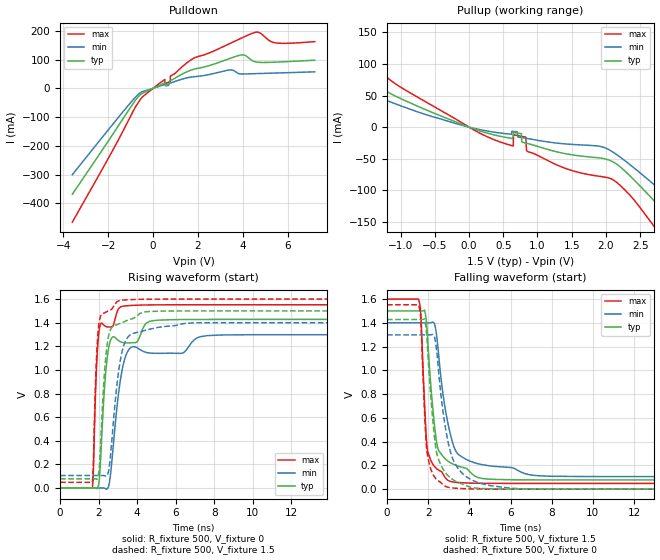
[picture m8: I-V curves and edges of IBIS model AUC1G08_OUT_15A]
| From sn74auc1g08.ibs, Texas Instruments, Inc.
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[Model]   AUC1G08_OUT_15A
Model_type  Output
Vref =   0
Rref =   2000
Cref =   15p
Vmeas =   0.75
| variable   typ   min   max
C_comp   7.20pF   2.74pF   16.84pF
| C_pullup   7.06pF   2.77pF   16.84pF
| C_pulldown   7.34pF   2.74pF   15.89pF
[Temperature Range]   40   100   -40
| Ambient temperature   25   85   -40
[Voltage range]   1.5   1.4   1.6
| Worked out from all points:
|   slope of the pulldown table from 0 to 0.225 V, typ, clamps not added: 27.2 ohm
|   slope of the pullup table from 0 to 0.225 V, typ, clamps not added: 27.6 ohm
|   rising waveform, R_fixture 500, V_fixture 0: 20-80 % time 361ps typ, 564ps min, 214ps max; typ from 0 V to 1.43 V
|   falling waveform, R_fixture 500, V_fixture 1.5: 20-80 % time 454ps typ, 736ps min, 255ps max; typ from 1.5 V to 0.078 V
|   rising waveform, R_fixture 500, V_fixture 1.5: 20-80 % time 344ps typ, 533ps min, 205ps max; typ from 0.078 V to 1.5 V
|   falling waveform, R_fixture 500, V_fixture 0: 20-80 % time 453ps typ, 701ps min, 256ps max; typ from 1.43 V to 0 V
[Pulldown]
| AUC1G08_OUT_15A
|   Voltage   I(typ)   I(min)   I(max)
-3.6V     -368.8mA   -300.6mA   -465.9mA
-570mV    -22.57mA   -15.16mA   -39.04mA
520mV     19.17mA    13.19mA    30.72mA
525mV     19.35mA    13.3mA     16.47mA
760mV     26.99mA    18.45mA    23.24mA
780mV     27.61mA    18.9mA     43.29mA
1.55V     59.04mA    37.1mA     91.54mA
3.425V    104mA      63.97mA    156.1mA
3.925V    116.2mA    49.97mA    174.5mA
4.58V     91.74mA    51.18mA    195.4mA
5.455V    91.13mA    53.24mA    158.3mA
7.2V      97.82mA    57.36mA    162.5mA
[Pullup]
| AUC1G08_OUT_15A
|   Voltage   I(typ)   I(min)   I(max)
-3.6V     253.4mA    202.6mA    313.9mA
-3.11V    208.7mA    165mA      264.9mA
-2.525V   156.9mA    121.3mA    206.3mA
-2.08V    119.5mA    90.68mA    162.1mA
80mV      -3.149mA   -2.07mA    -5.073mA
645mV     -8.448mA   -6.832mA   -29.87mA
830mV     -25.21mA   -17.58mA   -15.88mA
860mV     -25.98mA   -18.12mA   -38.83mA
2.065V    -52.94mA   -36.97mA   -81.25mA
2.79V     -126.2mA   -98.83mA   -169.6mA
3.55V     -215.2mA   -171.3mA   -279.9mA
7.2V      -643.1mA   -531.6mA   -796.6mA
[Ramp]
| AUC1G08_OUT_15A
| variable   typ   min   max
dV/dt_r   0.86/3.66E-10   0.79/5.70E-10   0.93/2.16E-10
dV/dt_f   0.86/4.64E-10   0.78/7.36E-10   0.93/2.56E-10
R_load = 500
[Rising Waveform]
| AUC1G08_OUT_15A
R_fixture =   500
C_fixture =   0
L_fixture =   0
V_fixture =   0
V_fixture_min = 0
V_fixture_max = 0
|   Time   V(typ)   V(min)   V(max)
0s        5.666nV    22.19nV    433.4pV
1.67ns    28.86uV    -4.974uV   968.1uV
1.88ns    -2.649mV   -6.943uV   995.4mV
2.035ns   79.02mV    138.4uV    1.346V
2.295ns   833.3mV    -1.097mV   1.375V
2.5ns     1.17V      7.839mV    1.363V
3.185ns   1.234V     972.6mV    1.537V
3.7ns     1.23V      1.193V     1.546V
7.63ns    1.427V     1.29V      1.552V
24.99ns   1.428V     1.298V     1.552V
[Falling Waveform]
| AUC1G08_OUT_15A
R_fixture =   500
C_fixture =   0
L_fixture =   0
V_fixture =   1.5
V_fixture_min = 1.4
V_fixture_max = 1.6
|   Time   V(typ)   V(min)   V(max)
0s        1.5V       1.4V       1.6V
1.54ns    1.5V       1.4V       1.594V
1.635ns   1.5V       1.4V       1.493V
1.83ns    1.502V     1.4V       691.6mV
1.965ns   1.293V     1.399V     325.6mV
2.42ns    384.1mV    1.279V     171.4mV
3.065ns   224.1mV    470.9mV    66.14mV
3.885ns   171.7mV    247.6mV    52.3mV
7.185ns   78.16mV    115.4mV    48.34mV
24.99ns   77.67mV    105.5mV    48.23mV
[Rising Waveform]
| AUC1G08_OUT_15A
R_fixture =   500
C_fixture =   0
L_fixture =   0
V_fixture =   1.5
V_fixture_min = 1.4
V_fixture_max = 1.6
|   Time   V(typ)   V(min)   V(max)
0s        77.64mV    105.5mV    48.22mV
1.67ns    77.67mV    105.5mV    50.4mV
1.87ns    76.02mV    105.5mV    1.041V
2.02ns    149.2mV    105.6mV    1.4V
2.265ns   889.4mV    105.2mV    1.48V
2.44ns    1.214V     106.5mV    1.495V
3.03ns    1.388V     983mV      1.584V
3.635ns   1.428V     1.297V     1.595V
6.49ns    1.5V       1.394V     1.6V
24.99ns   1.5V       1.4V       1.6V
[Falling Waveform]
| AUC1G08_OUT_15A
R_fixture =   500
C_fixture =   0
L_fixture =   0
V_fixture =   0
V_fixture_min = 0
V_fixture_max = 0
|   Time   V(typ)   V(min)   V(max)
0s        1.428V     1.298V     1.552V
1.535ns   1.428V     1.298V     1.548V
1.64ns    1.428V     1.298V     1.424V
1.82ns    1.433V     1.298V     666.8mV
1.955ns   1.229V     1.298V     294.6mV
2.37ns    346.1mV    1.222V     89.47mV
2.895ns   126.6mV    460.5mV    20.07mV
3.725ns   38.48mV    122.2mV    4.391mV
5.805ns   1.206mV    12mV       290.4uV
24.99ns   27.93uV    6.469uV    12.24uV
